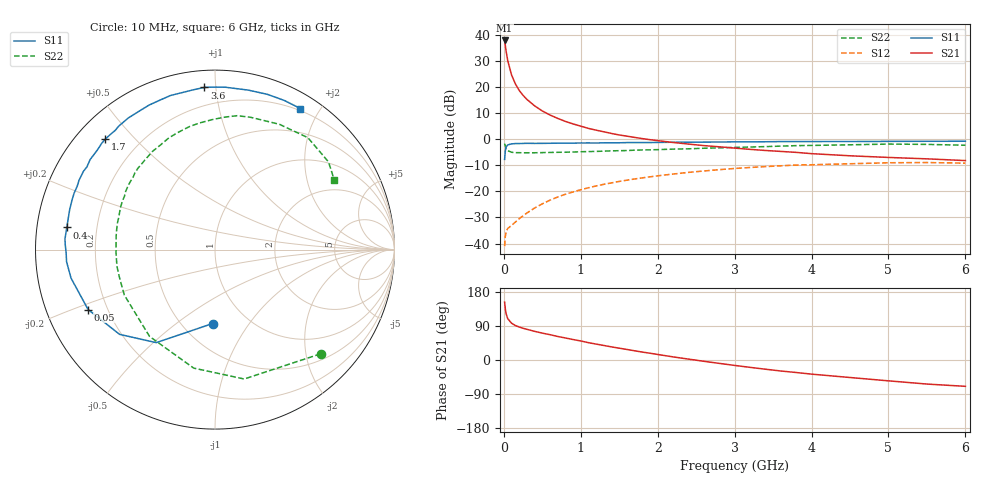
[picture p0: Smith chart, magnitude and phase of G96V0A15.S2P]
! SIEMENS Small Signal Semiconductors
! BFG235
! Si NPN RF Bipolar Junction Transistor in SOT223
! VCE = 6 V  IC = 150 mA
! Common Emitter S-Parameters:  July  1994
# GHz  S  MA  R  50
!  f  S11  S21  S12  S22
! GHz  MAG  ANG  MAG  ANG  MAG  ANG  MAG  ANG
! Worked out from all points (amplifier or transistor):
!   40 points, 10 MHz to 6 GHz, reference 50 ohm
!   highest |S21| = 37.9 dB at 10 MHz (marker M1)
!   |S21| within 3 dB of that: start of sweep to 24.46 MHz
!   unconditionally stable (mu >= 1): 457 MHz to 1.513 GHz
!   at 200 MHz: K = 0.80, MSG = 24.6 dB, |S12| = -30.5 dB
!   at 1.5 GHz: K = 1.00, MAG = 8.6 dB, |S12| = -16.2 dB
!   at 6 GHz: K = 0.89, MSG = 0.5 dB, |S12| = -9.2 dB
!   S11 on the Smith chart (normalised r, x): 10 MHz: 0.69, -0.69; 50 MHz: 0.13, -0.22; 400 MHz: 0.09, +0.07; 1.7 GHz: 0.08, +0.41; 3.6 GHz: 0.09, +0.93; 6 GHz: 0.17, +1.76
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0.01  0.412 -91.8  78.96 152.7  0.0089 63.3  0.8269 -44.6
0.02  0.6133 -122.3  62.25 133.8  0.014 48.2  0.739 -77.3
0.03  0.7111 -138.4  48.9 121.9  0.0168 41.3  0.6708 -100.2
0.05  0.7819 -154.7  32.64 109.3  0.0194 35.1  0.6058 -127.0
0.1  0.8177 -168.8  17.25 97.1  0.0222 37.4  0.5652 -153.4
0.15  0.8297 -175.3  11.59 91.0  0.0258 43.3  0.5543 -164.5
0.2  0.8296 -178.7  8.673 87.1  0.03 47.4  0.5542 -170.7
0.25  0.8346 178.2  6.986 83.7  0.0341 51.6  0.5513 -175.0
0.3  0.838 176.0  5.836 81.0  0.0385 54.3  0.5518 -178.6
0.4  0.835 171.5  4.391 75.6  0.0481 56.8  0.5522 176.2
0.5  0.8361 167.7  3.503 70.9  0.0578 58.0  0.5561 172.0
0.6  0.8399 164.5  2.926 66.8  0.068 58.2  0.5594 168.2
0.7  0.8429 161.0  2.523 62.1  0.0782 57.7  0.5636 164.7
0.9  0.8449 155.4  1.975 54.0  0.0979 55.0  0.5708 158.6
1.1  0.8529 149.3  1.62 45.7  0.1176 51.7  0.5825 152.4
1.7  0.8674 134.7  1.089 24.3  0.1736 39.5  0.6186 136.1
2.2  0.8781 123.4  0.87 8.2  0.2156 28.3  0.6483 122.5
3.2  0.8935 102.0  0.642 -19.4  0.288 5.2  0.7111 96.7
3.6  0.9055 93.8  0.586 -29.0  0.3103 -4.7  0.7402 85.7
4.5  0.9077 78.2  0.483 -46.2  0.3396 -24.6  0.785 62.8
5.5  0.9164 65.0  0.422 -63.5  0.3585 -46.5  0.7992 37.7
6  0.9189 58.8  0.391 -69.5  0.3487 -54.8  0.7698 30.4
